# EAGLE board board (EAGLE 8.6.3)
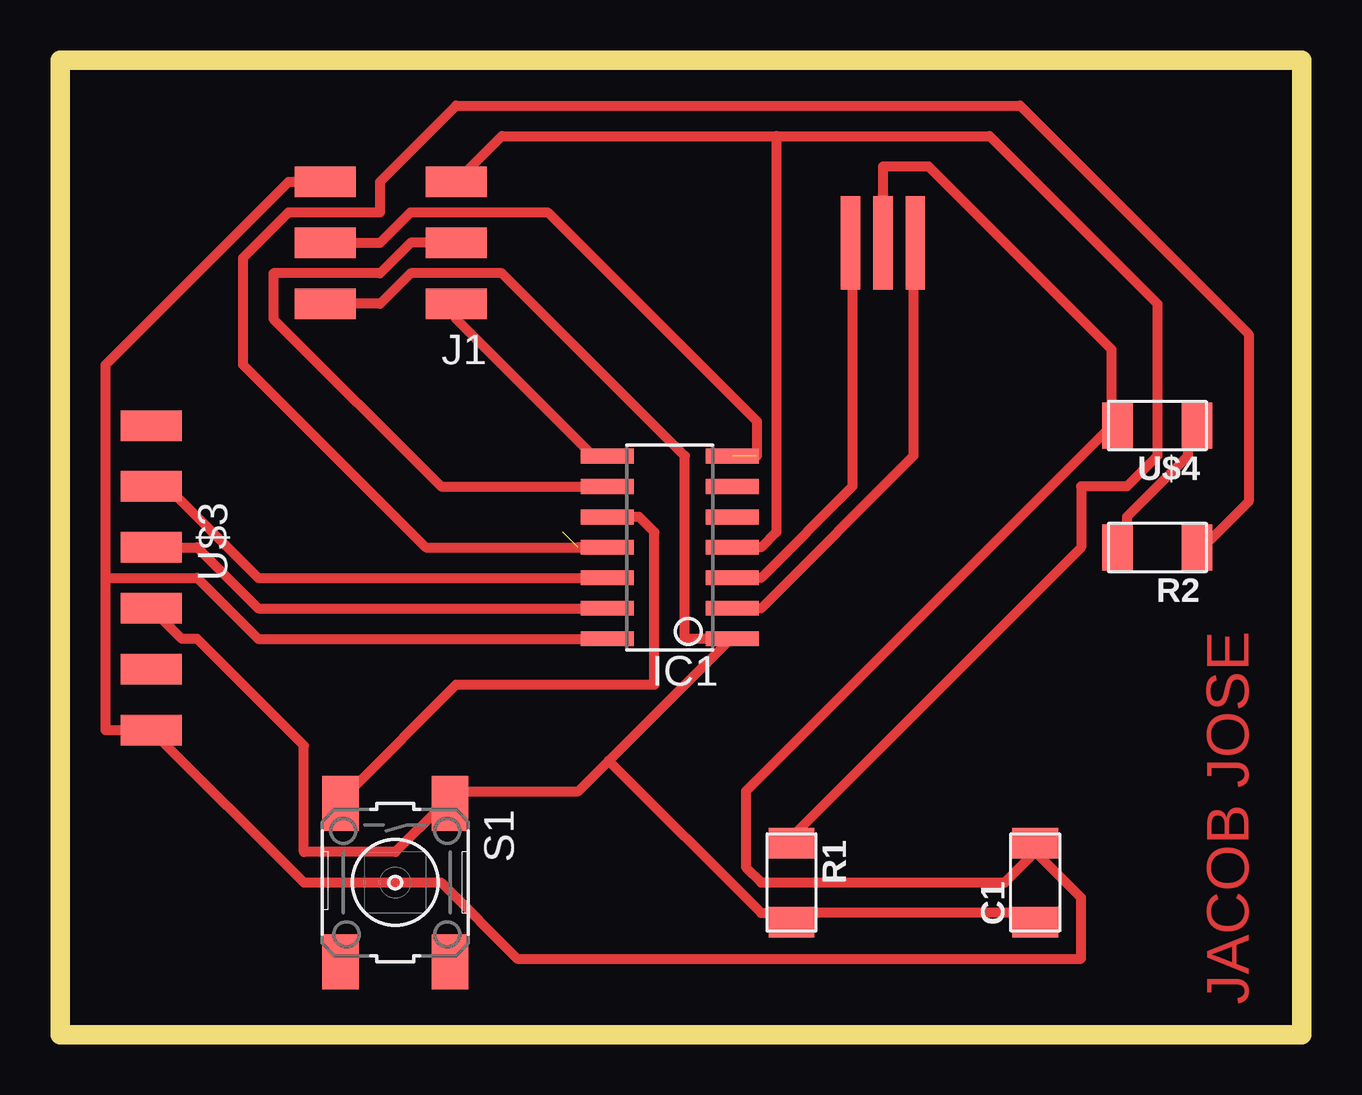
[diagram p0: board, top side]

Size 51.74 x 40.64 mm. Coordinates in mm from the lower left corner, seen from the top.
Outline: 0,0 51.74,0 51.74,40.63 0,40.64 0,0
Copper layers (1*16): Top 0.035mm / dielectric 1.5mm / Bottom 0.035mm
Design rules "default *": minimum track width 16mil, minimum drill 0.35mm, track to track 16mil, track to pad 16mil, pad to pad 16mil, via to via 16mil, smd to smd 16mil, copper to edge 40mil, drill to drill 16mil, minimum pad ring 10mil, minimum via ring 8mil, stop-mask expansion 4mil, vias tented up to drill 0mil, thermal gap 10mil
Net classes: 0 default: clearance 0.205 mm

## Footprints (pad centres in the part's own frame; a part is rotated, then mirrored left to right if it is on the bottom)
C1206FAB = smd 1.27 x 1.905: 1 -1.651,0; 2 1.651,0
SOIC14 = smd 0.61 x 2.21: 1 -3.81,-2.603; 2 -2.54,-2.603; 3 -1.27,-2.603; 4 0,-2.603; 5 1.27,-2.603; 6 2.54,-2.603; 7 3.81,-2.603; 8 3.81,2.603; 9 2.54,2.603; 10 1.27,2.603; 11 0,2.603; 12 -1.27,2.603; 13 -2.54,2.603; 14 -3.81,2.603
2X03SMD = smd 2.54 x 1.27: 1 -2.54,2.54; 2 2.92,2.54; 3 -2.54,0; 4 2.92,0; 5 -2.54,-2.54; 6 2.92,-2.54
R1206FAB = smd 1.27 x 1.905: 1 -1.651,0; 2 1.651,0
6MM_SWITCH = smd 2.286 x 1.524: 1 -3.302,2.286; 2 3.302,2.286; 3 -3.302,-2.286; 4 3.302,-2.286
1X06SMD = smd 2.54 x 1.27: 1 0,6.35; 2 0,3.81; 3 0,1.27; 4 0,-1.27; 5 0,-3.81; 6 0,-6.35
LED1206FAB = smd 1.27 x 1.905: 1 -1.651,0; 2 1.651,0
EFOBM = smd 0.8 x 3.9: 1 -1.35,0; 2 0,0; 3 1.35,0

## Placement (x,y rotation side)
C1  1µF  [C1206FAB]  40.64,6.35 90 top
IC1  ATTINY44-SSU  [SOIC14]  25.4,20.32 90 top
J1  AVRISPSMD  [2X03SMD]  13.97,33.02 180 top
R1  10K  [R1206FAB]  30.48,6.35 270 top
R2  499  [R1206FAB]  45.72,20.32 180 top
S1  [6MM_SWITCH]  13.97,6.35 270 top
U$3  FTDI-SMD-HEADER  [1X06SMD]  3.81,19.05 180 top
U$4  LEDFAB1206  [LED1206FAB]  45.72,25.4 180 top
XTAL1  RESONATOR  [EFOBM]  34.29,33.02 180 top

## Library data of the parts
C1 IC1 J1 R1 R2 S1 U$3 U$4 XTAL1 = fab

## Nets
GND: C1.2 IC1.14 J1.6 U$3.1 U$4.2 XTAL1.2
N$1: IC1.8 J1.1
N$2: IC1.7 J1.4
N$3: IC1.9 J1.3
N$4: IC1.12 U$3.5
N$5: IC1.13 U$3.4
N$6: IC1.3 XTAL1.3
N$7: IC1.2 XTAL1.1
N$8: IC1.4 J1.5 R1.1
N$9: R2.2 U$4.1
N$10: IC1.11 R2.1
N$11: IC1.10 S1.3
VCC: C1.1 IC1.1 J1.2 R1.2 S1.1 U$3.3

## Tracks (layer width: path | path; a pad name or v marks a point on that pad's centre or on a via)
GND
  Top 0.406: 40.64,7.62 39.37,6.35 29.21,6.35 28.57,6.98 28.57,10.16 43.82,25.4 | XTAL1.2 34.29,36.19 36.2,36.19 43.82,28.57 43.82,25.4 | 43.82,25.4 U$4.2 | IC1.14 8.26,16.51 5.71,19.05 1.9,19.05 | 1.9,19.05 1.9,12.7 U$3.1 10.16,6.35 15.88,6.35 19.05,3.18 42.54,3.18 42.54,5.71 40.64,7.62 | J1.6 9.52,35.56 1.9,27.94 1.9,19.05 | 40.64,7.62 C1.2
N$1
  Top 0.406: J1.1 16.51,29.85 22.23,24.13 IC1.8
N$2  (1 unrouted)
  Top 0.406: J1.4 13.34,33.02 14.6,34.29 20.32,34.29 29.03,25.58 29.03,24.13 | 27.94,24.13 IC1.7
N$3
  Top 0.406: IC1.9 15.88,22.86 8.89,29.85 8.89,31.75 13.34,31.75 14.6,33.02 J1.3
N$4
  Top 0.406: IC1.12 8.26,19.05 4.45,22.86 U$3.5
N$5
  Top 0.406: IC1.13 8.26,17.78 5.71,20.32 U$3.4
N$6
  Top 0.406: IC1.3 29.21,19.05 33.02,22.86 33.02,33.02 XTAL1.3
N$7
  Top 0.406: IC1.2 29.21,17.78 35.56,24.13 35.56,33.02 XTAL1.1
N$8
  Top 0.406: 29.84,37.47 18.41,37.47 J1.5 | R1.1 30.48,8.25 42.54,20.32 42.54,22.86 44.45,22.86 45.72,24.13 45.72,30.48 38.73,37.47 29.84,37.47 | IC1.4 29.21,20.32 29.84,20.96 29.84,37.47
N$9
  Top 0.406: R2.2 44.45,20.32 44.45,21.59 46.99,24.13 46.99,25.4 U$4.1
N$10  (1 unrouted)
  Top 0.406: 21.59,20.32 IC1.11 15.24,20.32 7.62,27.94 7.62,32.39 9.52,34.29 13.34,34.29 13.34,35.56 16.51,38.73 40.01,38.73 49.53,29.21 49.53,22.22 47.62,20.32 R2.1
N$11
  Top 0.406: IC1.10 24.13,21.59 24.77,20.96 24.77,14.61 16.51,14.61 12.06,10.16 S1.3
VCC
  Top 0.406: 30.48,5.08 40.64,5.08 C1.1 | 22.86,11.43 21.59,10.16 16.51,10.16 S1.1 15.88,9.52 13.97,7.62 10.16,7.62 10.16,12.06 5.71,16.51 5.08,16.51 U$3.3 | 22.86,11.43 27.94,16.51 | J1.2 13.34,30.48 14.6,31.75 18.41,31.75 26.03,24.13 26.03,16.51 27.94,16.51 | 27.94,16.51 IC1.1 | 30.48,5.08 29.21,5.08 22.86,11.43 | 30.48,5.08 R1.2

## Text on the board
Top: JACOB JOSE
